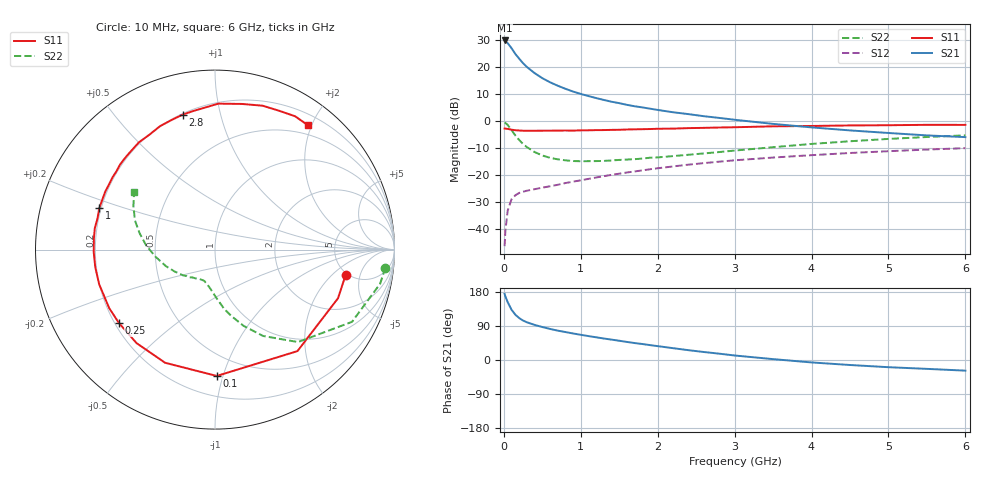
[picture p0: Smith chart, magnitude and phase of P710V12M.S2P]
! SIEMENS Small Signal Semiconductors
! BFP196
! Si NPN RF Bipolar Junction Transistor in SOT143
! VCE = 10 V  IC = 12 mA
! Common Emitter S-Parameters:  May  1996
# GHz  S  MA  R  50
!  f  S11  S21  S12  S22
! GHz  MAG  ANG  MAG  ANG  MAG  ANG  MAG  ANG
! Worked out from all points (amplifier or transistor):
!   36 points, 10 MHz to 6 GHz, reference 50 ohm
!   highest |S21| = 30.0 dB at 10 MHz (marker M1)
!   |S21| within 3 dB of that: start of sweep to 103.1 MHz
!   unconditionally stable (mu >= 1): 874.8 MHz to 3.43 GHz
!   at 250 MHz: K = 0.43, MSG = 23.8 dB, |S12| = -26.0 dB
!   at 1.4 GHz: K = 1.12, MAG = 11.4 dB, |S12| = -19.8 dB
!   at 6 GHz: K = 0.96, MSG = 2.0 dB, |S12| = -9.9 dB
!   S11 on the Smith chart (normalised r, x): 10 MHz: 4.76, -3.02; 100 MHz: 0.34, -0.95; 250 MHz: 0.22, -0.32; 1 GHz: 0.19, +0.17; 2.8 GHz: 0.21, +0.77; 6 GHz: 0.35, +1.95
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0.01  0.7414 -11.1  31.67 174.6  0.0049 81.7  0.9547 -6.1
0.02  0.737 -21.6  30.67 167.9  0.0094 77.6  0.9394 -11.7
0.05  0.7286 -50.9  28.24 152.6  0.0223 65.5  0.863 -27.8
0.1  0.7041 -89.2  22.77 132.7  0.0363 50.7  0.6922 -48.1
0.15  0.6891 -113.8  17.8 119.4  0.043 42.5  0.5507 -60.9
0.2  0.6801 -130.0  14.51 110.6  0.0475 37.7  0.4532 -69.5
0.25  0.6736 -142.6  12.01 104.1  0.05 35.4  0.3814 -76.1
0.3  0.6737 -151.0  10.21 99.5  0.0522 35.3  0.335 -81.1
0.4  0.6737 -163.3  7.869 92.6  0.0557 35.3  0.2715 -88.1
0.5  0.6743 -171.7  6.34 87.0  0.0594 36.4  0.2345 -93.7
0.6  0.6759 -178.9  5.328 82.0  0.0631 38.2  0.2123 -98.5
0.7  0.6776 174.6  4.598 77.5  0.0671 39.6  0.1991 -102.5
0.9  0.6773 165.0  3.582 70.0  0.0768 41.9  0.185 -108.4
1  0.6849 160.4  3.237 66.5  0.0813 43.0  0.1835 -111.2
1.1  0.6866 156.2  2.956 63.1  0.0864 43.7  0.184 -114.2
1.6  0.7102 138.2  2.032 47.7  0.1135 44.6  0.1971 -127.1
2.2  0.7371 119.8  1.482 31.2  0.147 41.8  0.2286 -141.1
2.8  0.7732 103.5  1.164 16.7  0.1801 36.6  0.2715 -156.9
3.5  0.8133 88.7  0.902 2.3  0.2147 29.3  0.3339 -173.2
4.5  0.8444 71.7  0.683 -13.2  0.2607 18.9  0.4302 167.7
5.5  0.8666 59.0  0.552 -23.4  0.3018 8.0  0.5157 151.8
6  0.8649 53.2  0.513 -28.1  0.3205 2.2  0.5536 144.5
